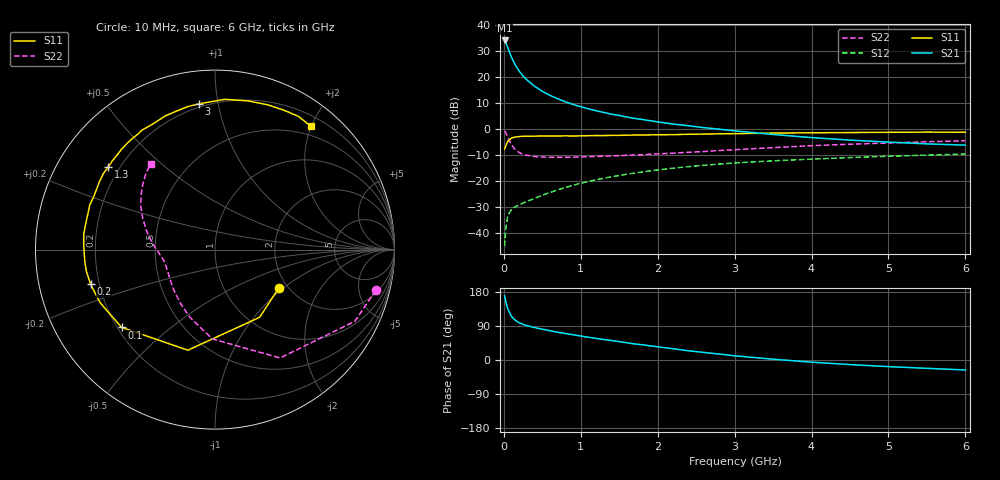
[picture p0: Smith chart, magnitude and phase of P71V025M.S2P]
! SIEMENS Small Signal Semiconductors
! BFP196
! Si NPN RF Bipolar Junction Transistor in SOT143
! VCE = 1 V  IC = 25 mA
! Common Emitter S-Parameters:  May  1996
# GHz  S  MA  R  50
!  f  S11  S21  S12  S22
! GHz  MAG  ANG  MAG  ANG  MAG  ANG  MAG  ANG
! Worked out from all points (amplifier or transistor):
!   36 points, 10 MHz to 6 GHz, reference 50 ohm
!   highest |S21| = 34.0 dB at 10 MHz (marker M1)
!   |S21| within 3 dB of that: start of sweep to 54.51 MHz
!   unconditionally stable (mu >= 1): 561.4 MHz to 5.098 GHz; 5.722 GHz to end of sweep
!   at 250 MHz: K = 0.68, MSG = 24.3 dB, |S12| = -28.4 dB
!   at 1.4 GHz: K = 1.12, MAG = 9.9 dB, |S12| = -18.3 dB
!   at 6 GHz: K = 1.01, MAG = 1.0 dB, |S12| = -9.6 dB
!   S11 on the Smith chart (normalised r, x): 10 MHz: 1.81, -0.92; 100 MHz: 0.22, -0.35; 200 MHz: 0.17, -0.13; 1.3 GHz: 0.16, +0.33; 3 GHz: 0.18, +0.88; 6 GHz: 0.35, +1.99
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0.01  0.4149 -30.7  49.93 169.5  0.0057 79.7  0.9239 -14.2
0.02  0.4518 -56.6  47.05 158.3  0.0109 71.0  0.876 -27.1
0.05  0.5805 -105.1  36.79 135.0  0.0215 52.2  0.7044 -59.0
0.1  0.6773 -140.2  23.62 114.7  0.029 42.2  0.4981 -91.7
0.15  0.7052 -155.2  16.75 104.5  0.0326 39.0  0.4024 -110.3
0.2  0.7194 -164.4  12.91 98.3  0.0352 40.7  0.3549 -123.1
0.25  0.7267 -170.4  10.38 94.0  0.0382 42.1  0.3282 -132.5
0.3  0.7285 -174.8  8.721 90.7  0.041 44.5  0.3142 -138.7
0.4  0.732 177.9  6.609 85.6  0.047 47.6  0.2976 -148.3
0.5  0.7364 173.2  5.295 81.3  0.0541 50.8  0.291 -154.5
0.6  0.7347 168.3  4.418 77.2  0.0609 52.4  0.2886 -158.6
0.7  0.7361 163.9  3.808 73.2  0.0684 53.7  0.2882 -161.7
0.9  0.7371 156.4  2.969 66.6  0.0839 54.5  0.2895 -166.7
1.1  0.7475 149.2  2.444 60.0  0.0992 53.9  0.2962 -170.1
1.3  0.7519 142.4  2.078 54.0  0.1145 52.5  0.302 -173.1
1.7  0.7683 129.5  1.601 42.4  0.1435 48.4  0.3185 -178.5
2.2  0.7813 116.0  1.25 29.6  0.1778 42.1  0.3451 175.3
3  0.8171 96.2  0.925 11.1  0.2242 31.1  0.402 163.3
3.5  0.839 86.3  0.788 2.1  0.2462 24.4  0.4413 156.1
4.5  0.8582 70.1  0.614 -12.1  0.2842 12.7  0.5129 143.3
5.5  0.8758 57.9  0.52 -22.0  0.3174 2.1  0.5717 132.4
6  0.8702 52.3  0.492 -26.3  0.3327 -3.7  0.5976 126.9
